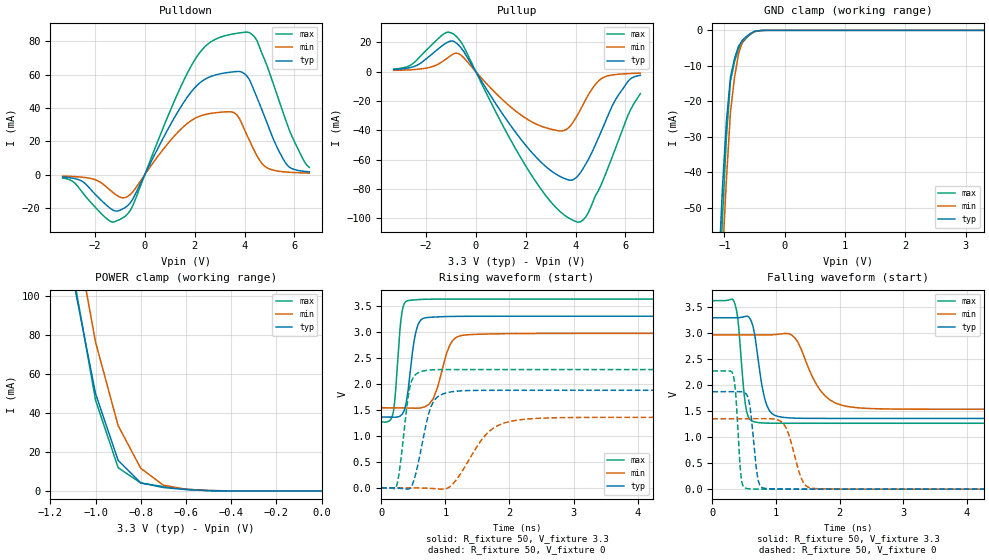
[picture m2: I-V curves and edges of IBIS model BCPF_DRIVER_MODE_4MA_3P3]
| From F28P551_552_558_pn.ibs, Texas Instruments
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|   Model Cell BCPF_DRIVER_MODE_4MA_3P3
|BCPF_DRIVER_MODE_4MA_3P3
[Model]   BCPF_DRIVER_MODE_4MA_3P3
Model_type   I/O
Polarity   Non-Inverting
Enable   Active-Low
Vinl =  0.8
Vinh =  2
Cref =  15.0000pF
Rref =  100.0000M
Vref =  0V
Vmeas =  1.65
C_comp   1.21982p   0.982413p   1.3757p
[Model Spec]
Vinl   0.8   0.8   0.8
Vinh   2   2   2
[Temperature Range]   25   155   -40
[Voltage Range]   3.3   2.97   3.63
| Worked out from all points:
|   slope of the pulldown table from 0 to 0.495 V, typ, clamps not added: 33.1 ohm
|   slope of the pullup table from 0 to 0.495 V, typ, clamps not added: 35.9 ohm
|   GND clamp passes 1 mA (typ) near -0.58 V on its own axis
|   POWER clamp passes 1 mA (typ) near -0.63 V on its own axis
|   rising waveform, R_fixture 50, V_fixture 3.3: 20-80 % time 123ps typ, 204ps min, 86.2ps max; typ from 1.36 V to 3.3 V
|   rising waveform, R_fixture 50, V_fixture 0: 20-80 % time 201ps typ, 444ps min, 132ps max; typ from 0 V to 1.88 V
|   falling waveform, R_fixture 50, V_fixture 3.3: 20-80 % time 149ps typ, 351ps min, 97.5ps max; typ from 3.3 V to 1.36 V
|   falling waveform, R_fixture 50, V_fixture 0: 20-80 % time 93.9ps typ, 189ps min, 68.1ps max; typ from 1.88 V to 0 V
| Nom Voltages:
|   BIASFET=3.3, VDD=1.2, VDDS=3.3, VSS=0
| Min Voltages:
|   BIASFET=2.97, VDD=1.08, VDDS=2.97, VSS=0
| Max Voltages:
|   BIASFET=3.63, VDD=1.32, VDDS=3.63, VSS=0
[POWER_clamp]
|   voltage   I(typ)   I(min)   I(max)
-3.3V     1.919A     2.431A     2.07A
-1.1V     109.5mA    140.7mA    112.6mA
-1.067V   89.71mA    119.3mA    90.66mA
-1.033V   69.89mA    97.95mA    68.7mA
-1V       50.07mA    76.56mA    46.74mA
-900mV    15.7mA     33.6mA     11.95mA
-800mV    4.139mA    11.64mA    4.053mA
-700mV    1.757mA    2.948mA    2.215mA
-600mV    692.2uA    840.1uA    875.7uA
-500mV    133.7uA    221.1uA    144.8uA
0V        61.4pA     4.167nA    15.35pA
[Pulldown]
|   voltage   I(typ)   I(min)   I(max)
-3.3V     -1.487mA   -922.6uA   -2.089mA
-2.5V     -4.195mA   -1.612mA   -10.83mA
-1.4V     -20.16mA   -9.277mA   -28.02mA
-800mV    -19.96mA   -13.89mA   -25.25mA
-500mV    -15.16mA   -10.71mA   -19.25mA
1.2V      34.55mA    23.42mA    44.71mA
2.1V      53.66mA    34.43mA    71.14mA
3.5V      61.62mA    37.57mA    84.38mA
4.1V      59.16mA    23.6mA     85.6mA
4.5V      46.26mA    11.27mA    80.53mA
5.6V      8.041mA    1.597mA    34.98mA
6.6V      1.614mA    874.2uA    4.301mA
[Pullup]
|   voltage   I(typ)   I(min)   I(max)
-3.3V     1.549mA    920.4uA    1.82mA
-2.6V     3.01mA     1.38mA     4.717mA
-1.8V     11.56mA    3.237mA    17.9mA
-900mV    20.89mA    12.22mA    25.89mA
-500mV    14.17mA    9.83mA     17.61mA
2.4V      -58.06mA   -35.58mA   -75.02mA
3.5V      -72.55mA   -40.32mA   -97.29mA
4.1V      -71.08mA   -28.84mA   -102.8mA
4.4V      -63.3mA    -19.25mA   -99.4mA
5V        -41.98mA   -5.103mA   -78.25mA
5.8V      -13.95mA   -1.59mA    -43.36mA
6.6V      -2.434mA   -956.3uA   -14.98mA
[GND_clamp]
|   voltage   I(typ)   I(min)   I(max)
-3.3V     -1.48A     -1.41A     -2.186A
-1.1V     -69.72mA   -89.95mA   -82.82mA
-1.033V   -44.46mA   -64.23mA   -52.87mA
-966.7mV  -25.61mA   -41.93mA   -30.06mA
-900mV    -13.19mA   -23.05mA   -14.39mA
-833.3mV  -7.976mA   -13.32mA   -8.853mA
-766.7mV  -4.491mA   -6.668mA   -5.2mA
-700mV    -2.738mA   -3.084mA   -3.432mA
-566.7mV  -869.7uA   -948.1uA   -1.077mA
-500mV    -261.7uA   -380.1uA   -295.9uA
-300mV    -598.3nA   -5.183uA   -296.7nA
3.3V      61.4pA     6.766uA    8.291pA
[Ramp]
| variable   typ   min   max
dV/dt_f  1.1815567/0.15050373n 0.87596502/0.35541151n  1.4353032/98.859284p
dV/dt_r  1.1402838/0.20374462n 0.82826393/0.44862262n  1.3772033/0.133218n
R_load = 50
[Rising Waveform]
R_fixture = 50
V_fixture = 3.3
V_fixture_min = 2.97
V_fixture_max = 3.63
|   time   V(typ)   V(min)   V(max)
0s        1.362V     1.539V     1.268V
172.6ps   1.358V     1.54V      1.381V
323.8ps   1.415V     1.538V     3.388V
389.4ps   1.641V     1.536V     3.588V
469.1ps   2.433V     1.532V     3.609V
627.2ps   3.24V      1.542V     3.624V
809.4ps   3.283V     1.713V     3.629V
1.109ns   3.296V     2.827V     3.63V
1.341ns   3.299V     2.944V     3.63V
20.01ns   3.3V       2.97V      3.63V
[Rising Waveform]
R_fixture = 50
V_fixture = 0
V_fixture_min = 0
V_fixture_max = 0
|   time   V(typ)   V(min)   V(max)
0s        0V         0V         0V
237.8ps   -3.226mV   0V         35.98mV
418.5ps   -23.96mV   0V         1.752V
479.5ps   45.07mV    0V         2.073V
725.7ps   1.362V     -7.201mV   2.263V
850.5ps   1.718V     -17.17mV   2.272V
1.035ns   1.834V     -2.972mV   2.275V
1.671ns   1.876V     1.076V     2.276V
2.429ns   1.876V     1.336V     2.275V
20.19ns   1.876V     1.355V     2.275V
[Falling Waveform]
R_fixture = 50
V_fixture = 3.3
V_fixture_min = 2.97
V_fixture_max = 3.63
|   time   V(typ)   V(min)   V(max)
0s        3.3V       2.97V      3.63V
344.8ps   3.3V       2.97V      3.602V
536.5ps   3.331V     2.97V      1.507V
641.7ps   3.119V     2.97V      1.303V
738.3ps   2.32V      2.969V     1.28V
964.5ps   1.432V     2.975V     1.27V
1.297ns   1.367V     2.912V     1.269V
1.845ns   1.363V     1.719V     1.269V
2.349ns   1.362V     1.561V     1.269V
20.01ns   1.362V     1.539V     1.269V
[Falling Waveform]
R_fixture = 50
V_fixture = 0
V_fixture_min = 0
V_fixture_max = 0
|   time   V(typ)   V(min)   V(max)
0s        1.876V     1.355V     2.275V
327ps     1.877V     1.355V     2.202V
454.2ps   1.876V     1.355V     208mV
582.9ps   1.643V     1.355V     7.102mV
724.1ps   151.1mV    1.357V     0V
877.8ps   9.642mV    1.358V     0V
1.119ns   2.278mV    1.258V     0V
1.43ns    0V         125.7mV    0V
1.619ns   0V         11.16mV    0V
20.19ns   0V         0V         0V
